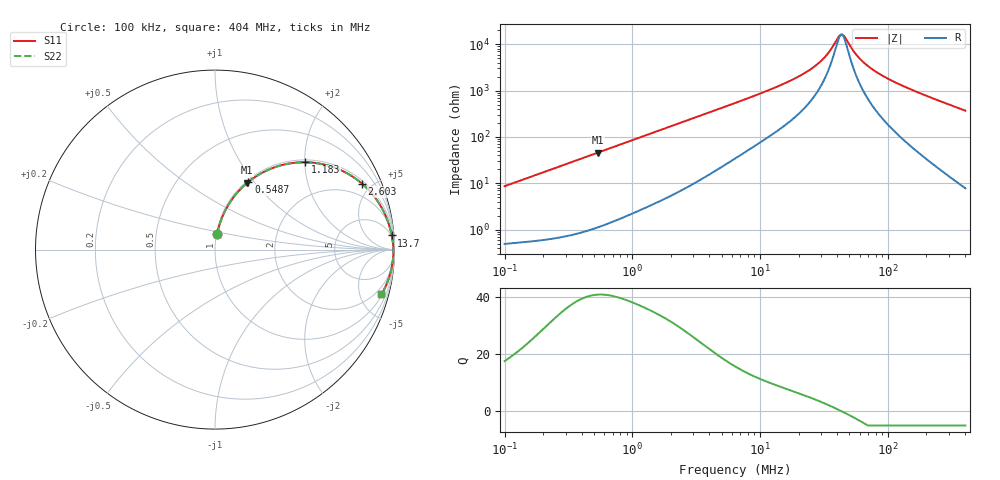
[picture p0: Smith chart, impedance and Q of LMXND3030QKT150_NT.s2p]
! LMXND3030QKT150_NT  S-PARAMETER MODEL  ( Standard Model )
! Model Generated by TAIYO YUDEN Corporation (https://www.yuden.co.jp/en/)
! Version 1.0
! TAIYO YUDEN Control No. 20250925
! Copyright(c) 2025 TAIYO YUDEN CO.,LTD. All Rights Reserved.
! Product Description (link to TY-COMPAS)
! https://ds.yuden.co.jp/TYCOMPAS/or/detail?pn=LMXND3030QKT150MNT&u=M
! Products Name : Inductors
! Characteristics :
!  Inductance : 15 [uH] , SRF(min) : 23 [MHz] , DC Resistance(max) : 0.39 [Ohm]
!  Rated Current : Saturation  580 [mA] , Temp Rise  930 [mA] (40 [degC])
!  Case Size : 3.0 x 3.0 / 0.118 x 0.118 [mm/inch] , Thickness : 1.5 / 0.059 [mm/inch]
!  (Conditions: Temperature = 25 [degC] , DC Bias Current = 0 [A])
! External Node Assignments :
!  1  o---GGG---o  2
! GND o---------o GND
! Frequency Range : 0.1MHz  -  403.964729MHz  [ 402 STEP ]
# MHz S RI R 50
! Freq[MHz].  S11 Real  S11 Imag  S21 Real  S21 Imag  S12 Real  S12 Imag  S22 Real  S22 Imag
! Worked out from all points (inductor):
!   401 points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, 100 kHz to 404 MHz, reference 50 ohm
!   read as one part in series: L = 13.7 uH near 104.2 kHz
!   highest Q = 40.9 at 537.4 kHz (marker M1), where L = 13.6 uH
!   self-resonance near 42.92 MHz
!   S11 on the Smith chart (normalised r, x): 100 kHz: 1.01, +0.17; 548.7 kHz: 1.02, +0.94; 1.183 MHz: 1.05, +2.01; 2.603 MHz: 1.16, +4.39; 13.7 MHz: 4, +24; 404 MHz: 1.16, -7.38
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0.1  0.0122 0.085  0.9878 -0.085  0.9878 -0.085  0.0122 0.085
0.202553  0.0348 0.1669  0.9652 -0.1669  0.9652 -0.1669  0.0348 0.1669
0.401849  0.1118 0.3028  0.8882 -0.3028  0.8882 -0.3028  0.1118 0.3028
0.537384  0.18 0.3722  0.82 -0.3722  0.82 -0.3722  0.18 0.3722
0.548656  0.186 0.3771  0.814 -0.3771  0.814 -0.3771  0.186 0.3771
1.182734  0.5016 0.4866  0.4984 -0.4866  0.4984 -0.4866  0.5016 0.4866
1.614823  0.6469 0.4634  0.3531 -0.4634  0.3531 -0.4634  0.6469 0.4634
2.603094  0.8196 0.3671  0.1804 -0.3671  0.1804 -0.3671  0.8196 0.3671
6.355822  0.9563 0.1752  0.0437 -0.1752  0.0437 -0.1752  0.9563 0.1752
13.7012  0.9847 0.0789  0.0153 -0.0789  0.0153 -0.0789  0.9847 0.0789
19.49971  0.9897 0.05  0.0103 -0.05  0.0103 -0.05  0.9897 0.05
25.54079  0.992 0.0316  0.00803 -0.0316  0.00803 -0.0316  0.992 0.0316
32.09288  0.9932 0.0175  0.00684 -0.0175  0.00684 -0.0175  0.9932 0.0175
41.17172  0.9938 0.00296  0.00616 -0.00296  0.00616 -0.00296  0.9938 0.00296
43.8174  0.9939 -0.000634  0.00608 0.000634  0.00608 0.000634  0.9939 -0.000634
46.63309  0.994 -0.00424  0.00603 0.00424  0.00603 0.00424  0.994 -0.00424
56.21301  0.9939 -0.0152  0.00608 0.0152  0.00608 0.0152  0.9939 -0.0152
63.66959  0.9937 -0.0228  0.00629 0.0228  0.00629 0.0228  0.9937 -0.0228
78.35931  0.993 -0.0364  0.007 0.0364  0.007 0.0364  0.993 -0.0364
102.6353  0.9912 -0.0563  0.00879 0.0563  0.00879 0.0563  0.9912 -0.0563
183.5443  0.9811 -0.1147  0.0189 0.1147  0.0189 0.1147  0.9811 -0.1147
403.9647  0.9271 -0.2497  0.0729 0.2497  0.0729 0.2497  0.9271 -0.2497
